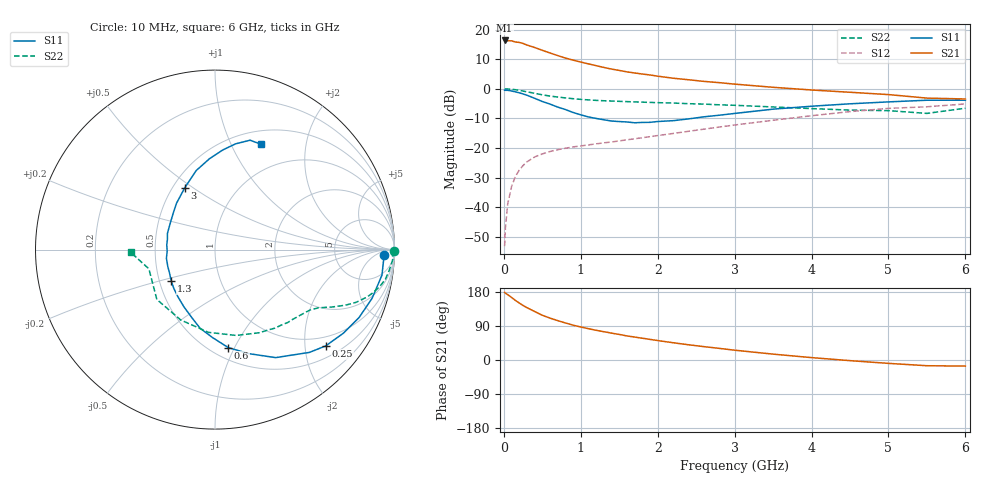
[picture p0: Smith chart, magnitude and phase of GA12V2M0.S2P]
! Infineon Technologies  Discrete & RF Semiconductors
! BF775
! Si NPN RF Bipolar Junction Transistor in SOT23
! VCE = 12 V  IC = 2 mA
! Common Emitter S-Parameters:  May  1996
# GHz  S  MA  R  50
!  f  S11  S21  S12  S22
! GHz  MAG  ANG  MAG  ANG  MAG  ANG  MAG  ANG
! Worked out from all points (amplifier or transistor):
!   36 points, 10 MHz to 6 GHz, reference 50 ohm
!   highest |S21| = 16.3 dB at 10 MHz (marker M1)
!   |S21| within 3 dB of that: start of sweep to 466.1 MHz
!   unconditionally stable (mu >= 1): 1.228 GHz to 3.111 GHz
!   at 250 MHz: K = 0.28, MSG = 20.6 dB, |S12| = -25.9 dB
!   at 1.4 GHz: K = 1.07, MAG = 10.7 dB, |S12| = -18.0 dB
!   at 6 GHz: K = 0.92, MSG = 0.8 dB, |S12| = -5.1 dB
!   S11 on the Smith chart (normalised r, x): 10 MHz: 27, -14; 250 MHz: 0.76, -2.47; 600 MHz: 0.60, -0.94; 1.3 GHz: 0.58, -0.22; 3 GHz: 0.57, +0.46; 6 GHz: 0.66, +1.31
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0.01  0.9432 -1.8  6.536 178.5  0.0022 85.3  0.9986 -0.6
0.02  0.9412 -3.5  6.408 176.6  0.0044 89.6  0.9896 -1.3
0.05  0.9411 -8.7  6.464 172.4  0.0113 85.2  0.9914 -3.4
0.1  0.9164 -17.2  6.44 165.2  0.0222 79.9  0.978 -6.7
0.15  0.8876 -25.2  6.159 157.3  0.033 75.3  0.9636 -9.9
0.2  0.8539 -33.0  6.057 150.5  0.0423 71.2  0.941 -12.6
0.25  0.8177 -41.0  5.817 143.9  0.0506 67.1  0.9134 -15.2
0.3  0.7779 -47.4  5.473 138.1  0.0583 64.1  0.8878 -17.3
0.4  0.6902 -60.7  4.972 128.0  0.0705 58.7  0.8389 -20.5
0.5  0.6089 -72.1  4.46 118.1  0.0794 54.5  0.7898 -23.1
0.6  0.5509 -82.3  4.017 110.5  0.0871 52.0  0.7522 -24.8
0.8  0.4456 -100.8  3.296 97.8  0.099 49.0  0.7003 -27.3
0.9  0.3976 -109.4  3.045 92.0  0.1043 48.6  0.6795 -28.4
1.1  0.3341 -128.3  2.63 82.7  0.1128 48.5  0.6481 -30.5
1.3  0.2995 -144.6  2.289 74.7  0.1222 49.1  0.627 -32.5
1.7  0.2665 -178.1  1.847 60.5  0.1429 51.1  0.5998 -37.5
2.2  0.289 149.8  1.506 45.6  0.1757 52.8  0.5737 -45.1
3  0.3829 116.2  1.197 25.9  0.2441 51.9  0.5258 -61.7
3.5  0.4526 103.4  1.058 15.5  0.2938 48.6  0.4927 -76.1
4.5  0.557 85.5  0.872 -1.7  0.4111 37.8  0.4362 -115.9
5.5  0.6401 72.2  0.695 -15.1  0.4963 21.1  0.3837 -163.8
6  0.6403 66.5  0.672 -16.1  0.5538 16.4  0.4694 -178.1
